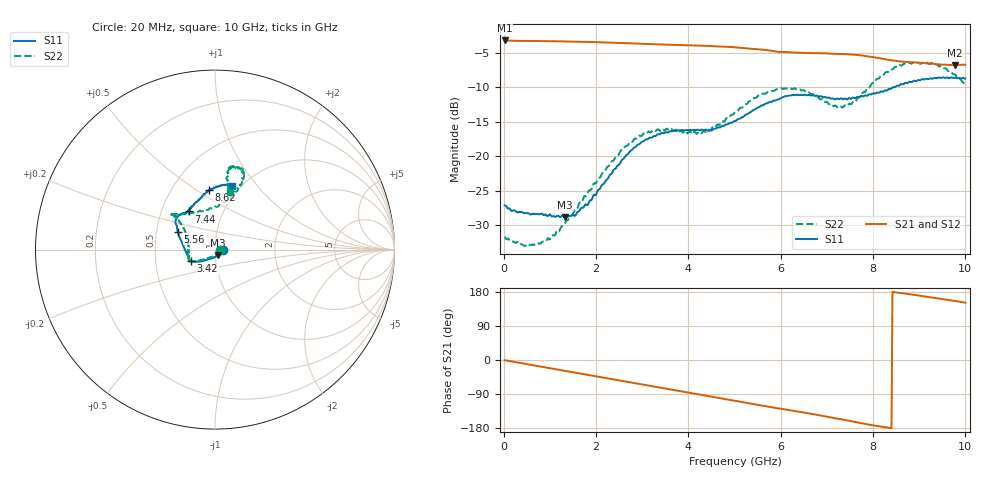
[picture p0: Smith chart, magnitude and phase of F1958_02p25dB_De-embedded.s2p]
! Integrated Device Technology
! Corporate Headquarters
! 6024 Silver Creek Valley Road
! San Jose, CA 95138  USA
! Phone:  1-408-284-8200
! Toll Free:  1-800-223-1366
! Webpage:  http://www.idt.com/
! Timing and RF Division
! 515 Groton Road, Suite 102
! Westford, MA 01886-6024
! Device:  F1958
! Description: 7-bit 0.25 dB Digital Step Attenuator
! Frequency:  0.001 -  6.000 GHz
! Package:  4x4 mm Thin QFN Plastic Package: 24 pin
! Ports:  2 RF, 12 DC
!  Pin  1  = D0
!  Pin  2  = VDD
!  Pin  3  = VMODE
!  Pin  4  = GND
!  Pin  5  = RF1  =  Port 1
!  Pin  6  = GND
!  Pin  7  = GND
!  Pin  8  = GND
!  Pin  9  = GND
!  Pin 10  = GND
!  Pin 11  = GND
!  Pin 12  = GND
!  Pin 13  = GND
!  Pin 14  = RF2  =  Port 2
!  Pin 15  = GND
!  Pin 16  = LE
!  Pin 17  = CLK
!  Pin 18  = DATA
!  Pin 19  = D6
!  Pin 20  = D5
!  Pin 21  = D4
!  Pin 22  = D3
!  Pin 23  = D2
!  Pin 24  = D1
! State:  9
! Atten State:  2.25 dB
! Voltage:  +3.30 Volts
! Current:  0.257 mA
! Data:  The device was measured on a F1958 evaluation board which has
!  individual transmission lines to the RF pins.  Data was collected
!  using a calibrated network analyzer.  The evaluation board was
!  de-embedded using Automatic Fixture Removal (AFR).
!  The reference plane is the edge of the package pin.
! Misc:
!  Action Tracker AT0419
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# GHz S dB R 50
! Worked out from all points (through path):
!   500 points, 20 MHz to 10 GHz, reference 50 ohm
!   highest |S21| = -3.23 dB at 20 MHz (marker M1); lowest = -6.8 dB at 9.78 GHz (marker M2)
!   group delay of S21, straight-line fit = 58.7 ps
!   lowest |S11| = -28.8 dB at 1.32 GHz (marker M3), VSWR 1.08, Z = 51.6 - j3.3 ohm
!   |S11| at or under -10 dB: start of sweep to 8.432 GHz; 8.456103 GHz to 8.467641 GHz (11.54 MHz wide, 0.136 % of centre)
!   |S22| runs from -33.0 to -6.4 dB; largest |S21 - S12| = 0.0018
!   S11 on the Smith chart (normalised r, x): 20 MHz: 1.09, -0.00; 3.42 GHz: 0.76, -0.10; 5.56 GHz: 0.64, +0.14; 7.44 GHz: 0.69, +0.31; 8.62 GHz: 0.75, +0.56; 10 GHz: 0.91, +0.74
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0.02  -27.12 -2.9  -3.23 -0.6  -3.23 -0.5  -31.67 -4.9
0.44  -28.23 -11.2  -3.29 -9.6  -3.29 -9.6  -32.94 -22.5
0.76  -28.40 -22.3  -3.31 -16.5  -3.31 -16.4  -32.59 -41.4
1.32  -28.83 -61.8  -3.37 -28.5  -3.37 -28.5  -29.85 -94.4
1.54  -28.65 -78.6  -3.40 -33.3  -3.40 -33.2  -27.83 -108.9
1.7  -27.43 -90.5  -3.43 -36.6  -3.42 -36.6  -26.54 -119.2
2.64  -19.93 -139.4  -3.61 -56.8  -3.60 -56.9  -18.52 -146.9
2.98  -17.95 -147.9  -3.70 -64.2  -3.69 -64.3  -17.09 -151.8
3.36  -16.81 -152.8  -3.80 -72.2  -3.80 -72.3  -16.21 -156.5
3.42  -16.60 -153.7  -3.81 -73.5  -3.81 -73.6  -16.07 -159.2
4.32  -16.22 -166.0  -3.98 -92.7  -4.00 -92.8  -16.34 171.8
5.02  -14.89 171.6  -4.22 -108.0  -4.23 -108.0  -13.51 146.2
5.56  -12.74 154.2  -4.53 -119.7  -4.55 -119.7  -11.21 140.8
6.02  -11.51 146.0  -4.88 -128.9  -4.90 -128.8  -10.16 140.8
6.68  -11.15 134.8  -5.06 -142.3  -5.07 -142.2  -11.00 134.9
7.2  -11.69 128.3  -5.17 -153.9  -5.18 -153.7  -12.66 110.9
7.44  -11.77 124.6  -5.23 -159.5  -5.24 -159.4  -12.76 93.0
8.34  -10.26 103.4  -6.04 -179.0  -6.04 -179.1  -7.69 67.9
8.62  -9.52 96.2  -6.27 176.4  -6.28 176.4  -6.85 70.3
9.28  -8.76 80.8  -6.60 164.6  -6.61 164.6  -6.51 79.2
9.78  -8.59 75.8  -6.79 155.8  -6.81 155.8  -8.16 79.6
10  -8.76 75.3  -6.74 151.2  -6.77 151.3  -9.63 75.4
